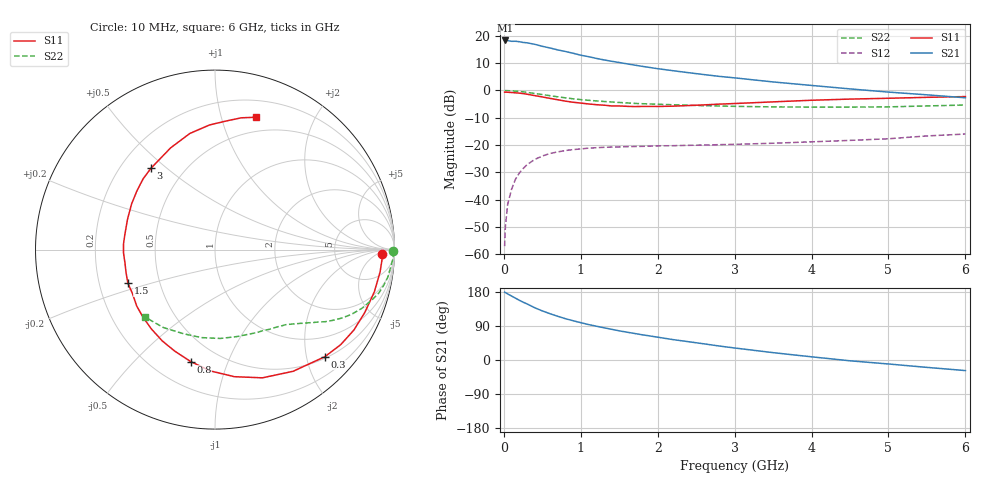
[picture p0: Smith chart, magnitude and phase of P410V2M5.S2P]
! SIEMENS Small Signal Semiconductors
! BFP182
! Si NPN RF Bipolar Junction Transistor in SOT143
! VCE = 10 V  IC = 2.5 mA
! Common Emitter S-Parameters:  March  1996
# GHz  S  MA  R  50
!  f  S11  S21  S12  S22
! GHz  MAG  ANG  MAG  ANG  MAG  ANG  MAG  ANG
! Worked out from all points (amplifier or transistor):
!   36 points, 10 MHz to 6 GHz, reference 50 ohm
!   highest |S21| = 18.3 dB at 20 MHz (marker M1)
!   |S21| within 3 dB of that: start of sweep to 634.2 MHz
!   unconditionally stable (mu >= 1): 2.123 GHz to end of sweep
!   at 250 MHz: K = 0.14, MSG = 23.1 dB, |S12| = -28.7 dB
!   at 1.4 GHz: K = 0.71, MSG = 15.7 dB, |S12| = -20.8 dB
!   at 6 GHz: K = 1.00, MAG = 6.3 dB, |S12| = -16.0 dB
!   S11 on the Smith chart (normalised r, x): 10 MHz: 26, -9; 300 MHz: 0.53, -2.36; 800 MHz: 0.35, -0.74; 1.5 GHz: 0.33, -0.17; 3 GHz: 0.33, +0.44; 6 GHz: 0.35, +1.30
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0.01  0.9334 -1.4  8.092 178.9  0.0014 82.7  0.9942 -0.6
0.02  0.9327 -3.1  8.259 178.1  0.0032 82.1  0.9941 -1.2
0.05  0.9283 -7.7  8.202 174.3  0.0082 88.6  0.9924 -3.1
0.1  0.9184 -14.9  7.969 168.9  0.0154 80.2  0.9823 -6.1
0.15  0.9051 -22.8  7.99 163.3  0.0234 76.7  0.9746 -9.2
0.2  0.8942 -30.1  7.836 157.8  0.0305 72.3  0.9605 -12.0
0.3  0.8551 -44.2  7.48 148.1  0.0435 65.0  0.9245 -17.1
0.4  0.8057 -57.3  7.032 138.0  0.0542 57.9  0.8824 -21.7
0.5  0.7617 -69.7  6.452 129.6  0.0629 52.0  0.8414 -25.4
0.6  0.7163 -81.3  6.011 122.2  0.07 46.6  0.8025 -28.4
0.7  0.6764 -92.2  5.544 115.4  0.0748 42.4  0.7654 -31.0
0.8  0.6381 -102.3  5.189 109.1  0.0793 38.6  0.7338 -33.2
0.9  0.6085 -111.6  4.814 103.6  0.0825 35.6  0.7031 -35.0
1.1  0.5662 -129.0  4.165 93.5  0.0877 30.6  0.6608 -38.1
1.5  0.5203 -158.8  3.256 77.0  0.0925 24.0  0.6027 -43.4
1.8  0.51 -177.9  2.769 66.5  0.0946 21.7  0.5723 -47.1
2.2  0.5159 160.9  2.303 53.8  0.0972 19.5  0.5471 -52.7
3  0.5766 128.3  1.703 31.7  0.103 18.3  0.5118 -65.9
3.5  0.6183 113.6  1.434 19.4  0.1079 17.9  0.5 -75.6
4.5  0.6952 92.5  1.069 -2.1  0.1217 17.5  0.496 -98.6
5.5  0.7488 78.7  0.832 -19.5  0.1468 16.8  0.5208 -123.5
6  0.7728 72.6  0.735 -27.9  0.159 13.8  0.5412 -135.9
